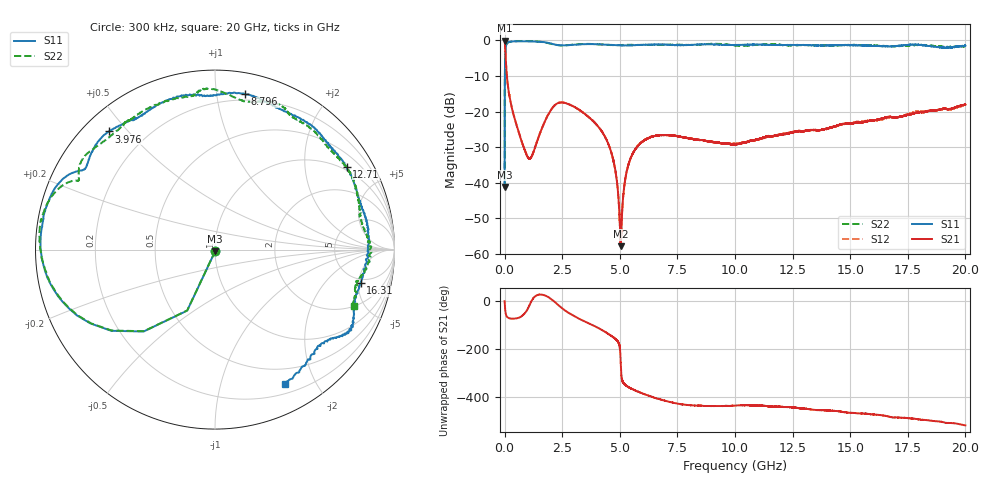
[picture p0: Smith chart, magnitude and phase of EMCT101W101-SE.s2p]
!EMCT101W101
!Johanson Technology Inc.
!www.johansontechnology.com
!Test Board Conditions:
!Substrate Type  RO4350B
!Substrate Thickness  10 mil
!Substrate Dk  3.66
!TL Type: GCPW
!TL Trace Width  22 mil
!TL Gap  14 mil
!PART MODE SINGLE ENDED (AKA BYPASS)
!DUT TOPOLOGY	SERIES-SHUNT
# MHz S  dB  R 50
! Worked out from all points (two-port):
!   20001 points, 300 kHz to 20 GHz, reference 50 ohm
!   highest |S21| = -0.02 dB at 1.3 MHz (marker M1); lowest = -57.8 dB at 5.044 GHz (marker M2)
!   |S21| within 3 dB of the highest: start of sweep to 30.8 MHz
!   lowest |S11| = -41.1 dB at 300 kHz (marker M3), VSWR 1.02, Z = 50.1 - j0.87 ohm
!   |S11| at or under -10 dB: start of sweep to 10.93 MHz
!   |S22| runs from -41.7 to -0.1 dB; largest |S21 - S12| = 0.0052
!   S11 on the Smith chart (normalised r, x): 300 kHz: 1.00, -0.02; 3.976 GHz: 0.07, +0.44; 8.796 GHz: 0.15, +1.20; 12.71 GHz: 0.87, +3.25; 16.31 GHz: 4.36, -5.31; 20 GHz: 0.30, -1.61
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0.3  -41.15 -81.9  -0.02 -0.6  -0.00 -0.6  -41.73 -84.1
1.3  -27.75 -92.2  -0.02 -2.4  -0.02 -2.4  -27.75 -92.1
101.298  -0.82 -163.1  -10.15 -65.7  -10.11 -65.7  -0.86 -162.8
124.298  -0.65 -166.4  -11.68 -68.0  -11.63 -68.1  -0.70 -166.0
408.294  -0.26 -179.6  -21.33 -73.5  -21.31 -73.7  -0.25 -179.2
1039.284  -0.23 168.3  -33.09 -26.3  -33.11 -25.9  -0.18 169.9
2192.267  -1.15 150.0  -18.14 -5.3  -18.07 -5.6  -1.20 153.8
3334.25  -1.09 139.2  -19.93 -78.8  -19.95 -78.8  -1.00 147.5
3976.24  -1.07 131.9  -23.54 -107.9  -23.54 -107.9  -1.04 141.7
4675.23  -1.27 124.6  -32.49 -148.3  -32.52 -148.5  -1.31 133.4
4835.227  -1.30 123.0  -37.71 -160.1  -37.72 -160.3  -1.33 131.1
5044.224  -1.38 122.2  -57.81 93.0  -57.26 92.8  -1.27 126.3
5263.221  -1.39 119.9  -38.00 9.2  -38.04 9.7  -1.27 125.4
5519.217  -1.36 117.1  -32.36 -5.1  -32.36 -4.6  -1.24 124.6
6667.2  -1.15 102.4  -26.71 -46.4  -26.69 -46.9  -1.21 118.6
8796.168  -1.09 79.0  -28.33 -76.5  -28.30 -76.8  -1.01 95.4
10000.15  -1.29 63.5  -29.18 -74.7  -29.00 -74.4  -1.37 82.2
12707.11  -1.24 32.2  -25.53 -84.4  -25.47 -84.7  -1.35 56.5
13334.1  -1.37 23.1  -25.21 -91.1  -25.16 -91.5  -1.34 47.9
16307.06  -1.59 -12.9  -22.08 -114.4  -22.28 -115.0  -1.48 16.7
16667.05  -1.67 -17.8  -21.50 -120.4  -21.72 -119.2  -1.61 13.4
20000  -1.44 -62.5  -18.00 -157.1  -18.13 -155.2  -1.60 -22.0
